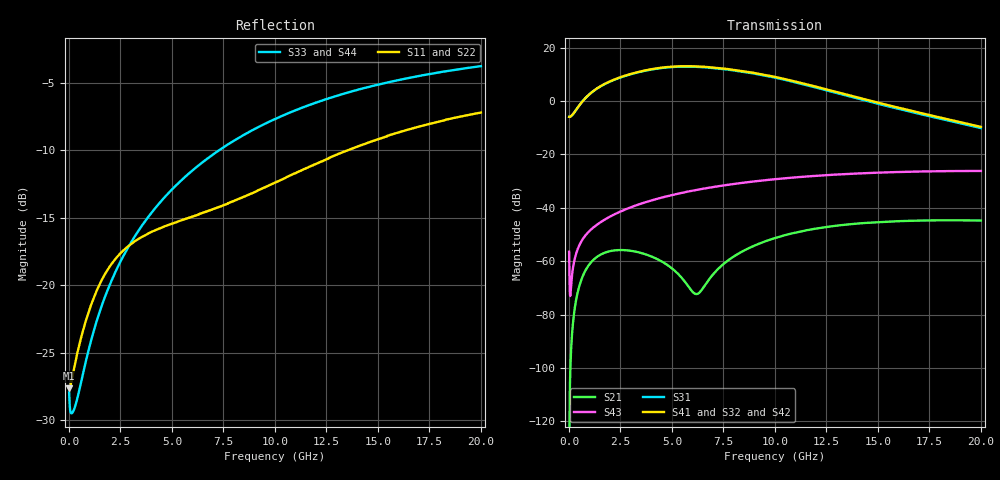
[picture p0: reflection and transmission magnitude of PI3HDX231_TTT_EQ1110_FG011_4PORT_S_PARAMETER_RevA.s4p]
! NPort=4 DATA=2000 NOISE=0 GROUPDELAY=0 COMPLEX_DATAFORMAT=POLAR
! NumOfBlock=1 NumOfParam=0
! .MODEL Smodel S TSTONEFILE=PI3HDX231_TTT_EQ1110_FG011_4PORT_S_PARAMETER_RevA.s4p TYPE=S
!  -- The above .MODEL line can be used for the S element in the netlist.
! The s parameter is extracted from the linear redriver, it is not bi-directional; only s(4,1)s(4,2) and s(3,1)s(3,2)
! should be the insertion loss
!Port definition:
!Port1 = input+
!Port2 = input-
!Port3 = output+
!Port4 = output-
# Hz S MA R  50
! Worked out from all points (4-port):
!   2000 points, 10 MHz to 20 GHz, reference 50 ohm
!   strongest paths, dB at 10 MHz, 5.01 GHz, 10.01 GHz, 15.01 GHz, 20 GHz:
!     S41: -5.9, 12.8, 9.0, -0.6, -9.7
!     S32: -5.9, 12.7, 8.9, -0.7, -9.7
!     S42: -5.9, 12.8, 8.9, -0.8, -9.8
!     S31: -5.9, 12.7, 8.7, -1.1, -10.1
!     S43: -56.5, -35.2, -29.3, -26.8, -26.2
!     S21: -134.8, -62.7, -51.3, -45.4, -44.8
!   lowest |S11| = -27.6 dB at 10 MHz (marker M1), VSWR 1.09, Z = 46 - j0.0776 ohm
!   |S11| at or under -10 dB: start of sweep to 13.55 GHz
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1e7  0.04152 -178.8  1.825e-07 -13.9  0 0.0  0 0.0
     1.825e-07 -14.0  0.04152 -178.8  0 0.0  0 0.0
     0.5043 0.4  0.5043 -179.6  0.04012 -3.2  0.0015 -70.3
     0.5043 -179.6  0.5043 0.4  0.0015 -70.3  0.04012 -3.2
3.27e9  0.1468 -140.8  0.001498 10.1  5.707e-11 -121.3  4.716e-11 -112.3
        0.0015 10.1  0.1468 -140.8  4.518e-11 -113.3  5.944e-11 -120.1
        3.374 -27.3  3.384 152.5  0.1548 -96.5  0.01114 69.9
        3.416 152.8  3.403 -26.5  0.01113 69.8  0.1548 -96.5
5.32e9  0.1724 -139.5  0.0005633 -10.5  1.024e-09 172.9  7.08e-10 -163.9
        0.0005672 -10.4  0.1723 -139.7  6.688e-10 -163.3  1.08e-09 173.0
        4.381 -92.8  4.402 87.1  0.2389 -103.4  0.01849 59.8
        4.454 87.0  4.438 -92.0  0.01844 59.7  0.239 -103.4
7.49e9  0.1977 -134.7  0.0008819 103.0  7.308e-09 106.6  5.328e-09 139.4
        0.000875 102.5  0.1972 -134.9  5.09e-09 141.4  7.694e-09 105.5
        3.962 -161.0  4.004 18.8  0.3233 -109.4  0.02624 46.8
        4.052 18.5  4.024 -160.1  0.02615 46.8  0.3235 -109.4
1.012e10  0.2419 -129.5  0.002813 84.1  3.451e-08 32.6  2.701e-08 64.5
          0.002797 83.8  0.2407 -129.6  2.632e-08 67.1  3.585e-08 30.6
          2.676 125.8  2.734 -54.6  0.4161 -116.0  0.03471 29.8
          2.76 -55.2  2.727 126.8  0.03461 29.9  0.4162 -116.0
1.328e10  0.3098 -128.3  0.004787 50.9  1.074e-07 -42.3  8.546e-08 -16.7
          0.004758 50.6  0.3078 -128.3  8.501e-08 -14.1  1.095e-07 -44.6
          1.318 54.8  1.37 -126.5  0.5094 -123.0  0.04254 9.1
          1.375 -127.3  1.35 55.9  0.04249 9.4  0.5093 -123.1
2e10  0.4356 -135.6  0.005809 -4.0  3.764e-07 -162.6  2.826e-07 -146.1
      0.005766 -4.1  0.4339 -135.4  2.867e-07 -144.6  3.76e-07 -164.4
      0.3112 -50.9  0.3289 124.0  0.6464 -135.0  0.04883 -32.3
      0.327 123.5  0.3222 -49.9  0.04896 -32.1  0.6461 -135.0
